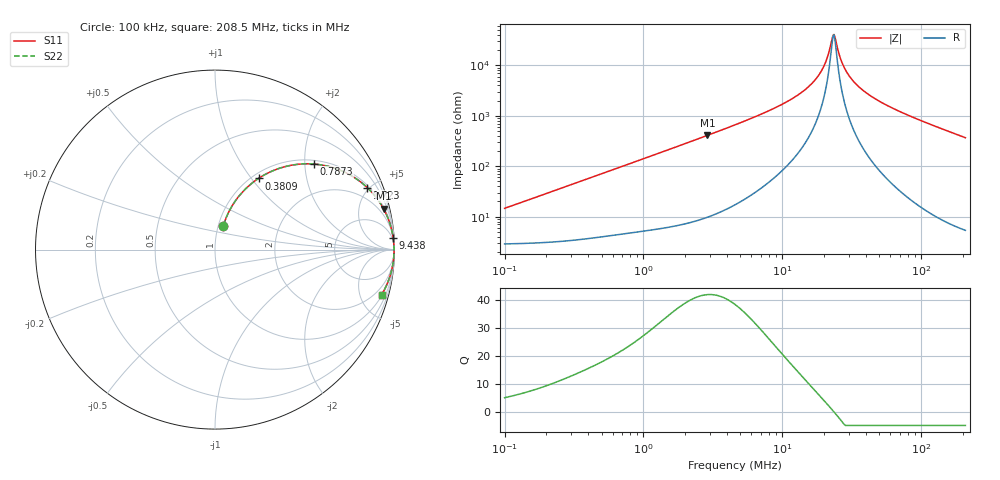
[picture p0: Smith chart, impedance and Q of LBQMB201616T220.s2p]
! LBQMB201616T220  S-PARAMETER MODEL  ( General Type )
! Model Generated by TAIYO YUDEN Corporation (http://www.ty-top.com)
! Version 1.0
! TAIYO YUDEN Control No. 191025NI43SB-FBB
! Copyright(c) 2019 TAIYO YUDEN CO.,LTD. All Rights Reserved.
! Product Description (link to TY-COMPAS)
! https://ds.yuden.co.jp/TYCOMPAS/or/detail?pn=LBQMB201616T220J&u=M
! Products Name : Inductors
! Characteristics :
!  Inductance : 22 uH , SRF(min) : 17 MHz , DC Resistance(max) : 3.64 Ohm , Rated Current : 140 mA
!  Case Size : 2.0 x 1.6 / 0.079 x 0.063 [mm/inch] , Thickness : 1.6 / 0.063 [mm/inch]
!  (Conditions: Temperature = 25 degC , DC Bias Current/Voltage = 0A / 0V)
! External Node Assignments :
!  1  o---GGG---o  2
! GND o---------o GND
! Frequency Range : 0.1MHz  -  208.503118MHz  [ 402 STEP ]
# MHz S RI R 50
! Freq[MHz].  S11 Real  S11 Imag  S21 Real  S21 Imag  S12 Real  S12 Imag  S22 Real  S22 Imag
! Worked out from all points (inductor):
!   401 points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, 100 kHz to 208.5 MHz, reference 50 ohm
!   read as one part in series: L = 22.8 uH near 103.9 kHz
!   highest Q = 42.1 at 2.887 MHz (marker M1), where L = 22.5 uH
!   self-resonance near 23.17 MHz
!   S11 on the Smith chart (normalised r, x): 100 kHz: 1.06, +0.29; 380.9 kHz: 1.07, +1.08; 787.3 kHz: 1.09, +2.22; 1.723 MHz: 1.13, +4.85; 9.438 MHz: 2, +31; 208.5 MHz: 1.11, -7.36
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0.1  0.0465 0.133  0.9535 -0.133  0.9535 -0.133  0.0465 0.133
0.206688  0.1038 0.2571  0.8962 -0.2571  0.8962 -0.2571  0.1038 0.2571
0.359709  0.2242 0.3839  0.7758 -0.3839  0.7758 -0.3839  0.2242 0.3839
0.38093  0.2424 0.3965  0.7576 -0.3965  0.7576 -0.3965  0.2424 0.3965
0.787337  0.5505 0.4767  0.4495 -0.4767  0.4495 -0.4767  0.5505 0.4767
1.293906  0.761 0.411  0.239 -0.411  0.239 -0.411  0.761 0.411
1.723334  0.8478 0.3458  0.1522 -0.3458  0.1522 -0.3458  0.8478 0.3458
2.886752  0.9388 0.2281  0.0612 -0.2281  0.0612 -0.2281  0.9388 0.2281
4.654297  0.975 0.1437  0.025 -0.1437  0.025 -0.1437  0.975 0.1437
9.437826  0.9931 0.0632  0.00689 -0.0632  0.00689 -0.0632  0.9931 0.0632
13.05973  0.9959 0.0377  0.00411 -0.0377  0.00411 -0.0377  0.9959 0.0377
16.42508  0.9969 0.0222  0.00306 -0.0222  0.00306 -0.0222  0.9969 0.0222
19.88316  0.9974 0.0102  0.00258 -0.0102  0.00258 -0.0102  0.9974 0.0102
21.05614  0.9975 0.00665  0.00249 -0.00665  0.00249 -0.00665  0.9975 0.00665
22.72846  0.9976 0.00197  0.00242 -0.00197  0.00242 -0.00197  0.9976 0.00197
23.61378  0.9976 -0.000368  0.0024 0.000368  0.0024 0.000368  0.9976 -0.000368
24.06929  0.9976 -0.00154  0.00239 0.00154  0.00239 0.00154  0.9976 -0.00154
27.51362  0.9976 -0.00976  0.00243 0.00976  0.00243 0.00976  0.9976 -0.00976
31.45084  0.9974 -0.0182  0.00261 0.0182  0.00261 0.0182  0.9974 -0.0182
40.31841  0.9966 -0.0348  0.00341 0.0348  0.00341 0.0348  0.9966 -0.0348
59.08252  0.9936 -0.0649  0.00639 0.0649  0.00639 0.0649  0.9936 -0.0649
208.5031  0.9282 -0.251  0.0718 0.251  0.0718 0.251  0.9282 -0.251
